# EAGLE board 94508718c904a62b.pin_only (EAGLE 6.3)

Size 17.78 x 37.34 mm. Coordinates in mm from the lower left corner, seen from the top.
Outline: 17.78,1.72 17.78,35.43 arc90 15.88,37.34 1.91,37.34 arc90 0,35.43 0,1.27 1.14,1.27 2.41,0 11.62,0 12.89,1.27 17.4,1.27 17.78,1.72
Copper layers (1*16): Top 0.035mm / dielectric 1.5mm / Bottom 0.035mm
Design rules "adafruit": minimum track width 8mil, minimum drill 15.5mil, track to track 8mil, track to pad 8mil, pad to pad 8mil, via to via 8mil, smd to smd 8mil, copper to edge 10mil, drill to drill 8mil, minimum pad ring 10mil, minimum via ring 8mil, stop-mask expansion 2mil, vias tented up to drill 20mil, thermal gap 10mil
Net classes: 1 power: width 0.305 mm
Holes 2.2 mm at 1.91,35.56 15.88,35.56 8.89,9.78

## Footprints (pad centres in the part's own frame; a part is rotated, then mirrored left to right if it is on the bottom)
CHIPLED_0805_NOOUTLINE = smd 1.2 x 1.2: A 0,-1.05; C 0,1.05
JSTPH2 = smd 1 x 4.6: 1 -1,-3.7; 2 1,-3.7 | smd 1.6 x 3.4: NC1 -3.4,1.5; NC2 3.4,1.5
0805-NO = smd 1.3 x 1.5: 1 -0.95,0; 2 0.95,0
_0805MP = smd 1.2 x 1.3: 1 -1.016,0; 2 1.016,0
4UCONN_20329 = smd 1 x 2: BASE@1 -0.75,-2; BASE@2 0.75,-2 | smd 0.4 x 1.35: D+ 0,0.775; D- -0.65,0.775; GND 1.3,0.775; ID 0.65,0.775; VBUS -1.3,0.775 | drill 0.7 offset: SPRT@1 -3.3,0.9; SPRT@2 3.3,0.9 | drill 0.6 pad 2.5 square: SPRT@3 -3.6,-1.9; SPRT@4 3.6,-1.9 | hole 0.7: -1.95,0; 1.95,0
SOD-323 = smd 1.35 x 0.8: A 1.27,0; C -1.27,0
SOD-123FL = smd 0.91 x 1.22: A 1.637,0; C -1.637,0
1X06-CLEANBIG = drill 1.016 pad 1.778 octagon: 1 -6.35,0; 2 -3.81,0; 3 -1.27,0; 4 1.27,0; 5 3.81,0; 6 6.35,0
MLF32-TH = smd 0.7 x 0.25: 1 -2.35,1.75; 2 -2.35,1.25; 3 -2.35,0.75; 4 -2.35,0.25; 5 -2.35,-0.25; 6 -2.35,-0.75; 7 -2.35,-1.25; 8 -2.35,-1.75; 17 2.35,-1.75; 18 2.35,-1.25; 19 2.35,-0.75; 20 2.35,-0.25; 21 2.35,0.25; 22 2.35,0.75; 23 2.35,1.25; 24 2.35,1.75 | smd 0.25 x 0.7: 9 -1.75,-2.35; 10 -1.25,-2.35; 11 -0.75,-2.35; 12 -0.25,-2.35; 13 0.25,-2.35; 14 0.75,-2.35; 15 1.25,-2.35; 16 1.75,-2.35; 25 1.75,2.35; 26 1.25,2.35; 27 0.75,2.35; 28 0.25,2.35; 29 -0.25,2.35; 30 -0.75,2.35; 31 -1.25,2.35; 32 -1.75,2.35 | smd 3.2 x 3.2: TH 0,0
SOT23-5L = smd 0.55 x 1.2: 1 -0.95,-1.3; 2 0,-1.3; 3 0.95,-1.3; 4 0.95,1.3; 5 -0.95,1.3
1X12-CB = drill 1.016 pad 1.778: 1 -13.97,0; 2 -11.43,0; 3 -8.89,0; 4 -6.35,0; 5 -3.81,0; 6 -1.27,0; 7 1.27,0; 8 3.81,0; 9 6.35,0; 10 8.89,0; 11 11.43,0; 12 13.97,0
1X02_ROUND = drill 1 pad 1.778: 1 -1.27,0; 2 1.27,0
BTN_KMR2_4.6X2.8 = smd 0.9 x 1: A 2.05,0.8; A' -2.05,0.8; B 2.05,-0.8; B' -2.05,-0.8
0603-NO = smd 1.1 x 1: 1 -0.85,0; 2 0.85,0
FIDUCIAL_1MM = smd 1 x 1: 1 0,0
RESONATOR-SMD = smd 0.7 x 1.7: 1 -1.2,0; 2 0,0; 3 1.2,0

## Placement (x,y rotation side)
B1  red  [CHIPLED_0805_NOOUTLINE]  6.73,30.23 270 top
BAT  JST 2-PH  [JSTPH2]  8.89,33.78 0 bottom
C1  10uF  [0805-NO]  5.46,22.73 270 top
C2  0.1uF  [_0805MP]  4.32,19.56 0 top
C3  0.1uF  [0805-NO]  12.7,6.86 270 top
C8  10uF  [0805-NO]  11.91,22.35 270 top
CN1  [4UCONN_20329]  8.89,33.02 180 top
D1  3.6v  [SOD-323]  5.21,26.92 90 top
D2  SCHOTTKY  [SOD-123FL]  12.57,26.49 90 top
D4  3.6V  [SOD-323]  10.79,26.42 270 top
FTDI  [1X06-CLEANBIG]  8.89,2.54 0 top
IC1  ATmega328P  [MLF32-TH]  8.89,15.37 180 top
IC2  MIC5225-5v  [SOT23-5L]  9.02,22.48 270 top
JP1  [1X12-CB]  16.51,19.05 270 top
JP2  [1X02_ROUND]  3.81,16.51 270 top
JP4  [1X12-CB]  1.27,19.05 270 top
PWR  green  [CHIPLED_0805_NOOUTLINE]  11.56,30.29 90 top
Q1  reset  [BTN_KMR2_4.6X2.8]  8.89,6.35 0 top
R1  68 (0603)  [0603-NO]  8,26.8 270 top
R2  68 (0603)  [0603-NO]  6.73,26.8 270 top
R3  1.5K (0603)  [0603-NO]  9.4,26.8 270 top
R4  470 (0603)  [0603-NO]  13.97,28.83 270 top
R5  470 (0603)  [0603-NO]  4.06,29.59 270 top
R6  10K  [0805-NO]  5.33,6.6 270 top
U$1  FIDUCIAL  [FIDUCIAL_1MM]  14.48,24 0 top
U$6  FIDUCIAL  [FIDUCIAL_1MM]  8.89,6.35 0 top
U$7  [ADAFRUIT_3.5MM]  4.06,8.51 0 top
U$9  [ADAFRUIT_9MM]  5.33,9.53 90 bottom
Y1  16MHz  [RESONATOR-SMD]  13.46,16.89 90 top

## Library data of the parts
B1 BAT C1-C3 C8 CN1 D1 D4 JP2 PWR Q1 R1-R6 U$7 U$9 = microbuilder
D2 FTDI IC2 JP1 JP4 U$1 U$6 = adafruit
IC1 = microbuilder; MPN: ATMEGA88PA-MU; OC_FARNELL: 1715491; OC_NEWARK: 15R0272
Y1 = SparkFun

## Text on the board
tPlace: + | 9 | ~ | ~ | BAT | G | 10 | 11 | pwr | BUS | ~ | #13 | 12 | 5V | 13 | 8 | Ar | Pro | 6 | ~ | Trinket! | 5 | ~ | A6 | A0 | 4 | A1 | A7 | 16 / MHz | ~ | A2 | 3 | A3 | 5V | TX | A4 | RX | RST | A5 | BLK | GND | 5V | RX | TX | GRN | FTDI Header
bPlace: VBat / JST | + | - | Adafruit / Pro Trinket / ATmega328p / 5V / 16MHz | VBat: 5-16VDC | USBtinyISP / or UNO FTDI / Bootloader

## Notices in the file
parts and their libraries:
microbuilder: This work is placed in the public domain, and may be freely used for commercial and non-commercial work with the following conditions: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
SparkFun: Licensing: CC v3.0 Share-Alike You are welcome to use this library for commercial purposes.
